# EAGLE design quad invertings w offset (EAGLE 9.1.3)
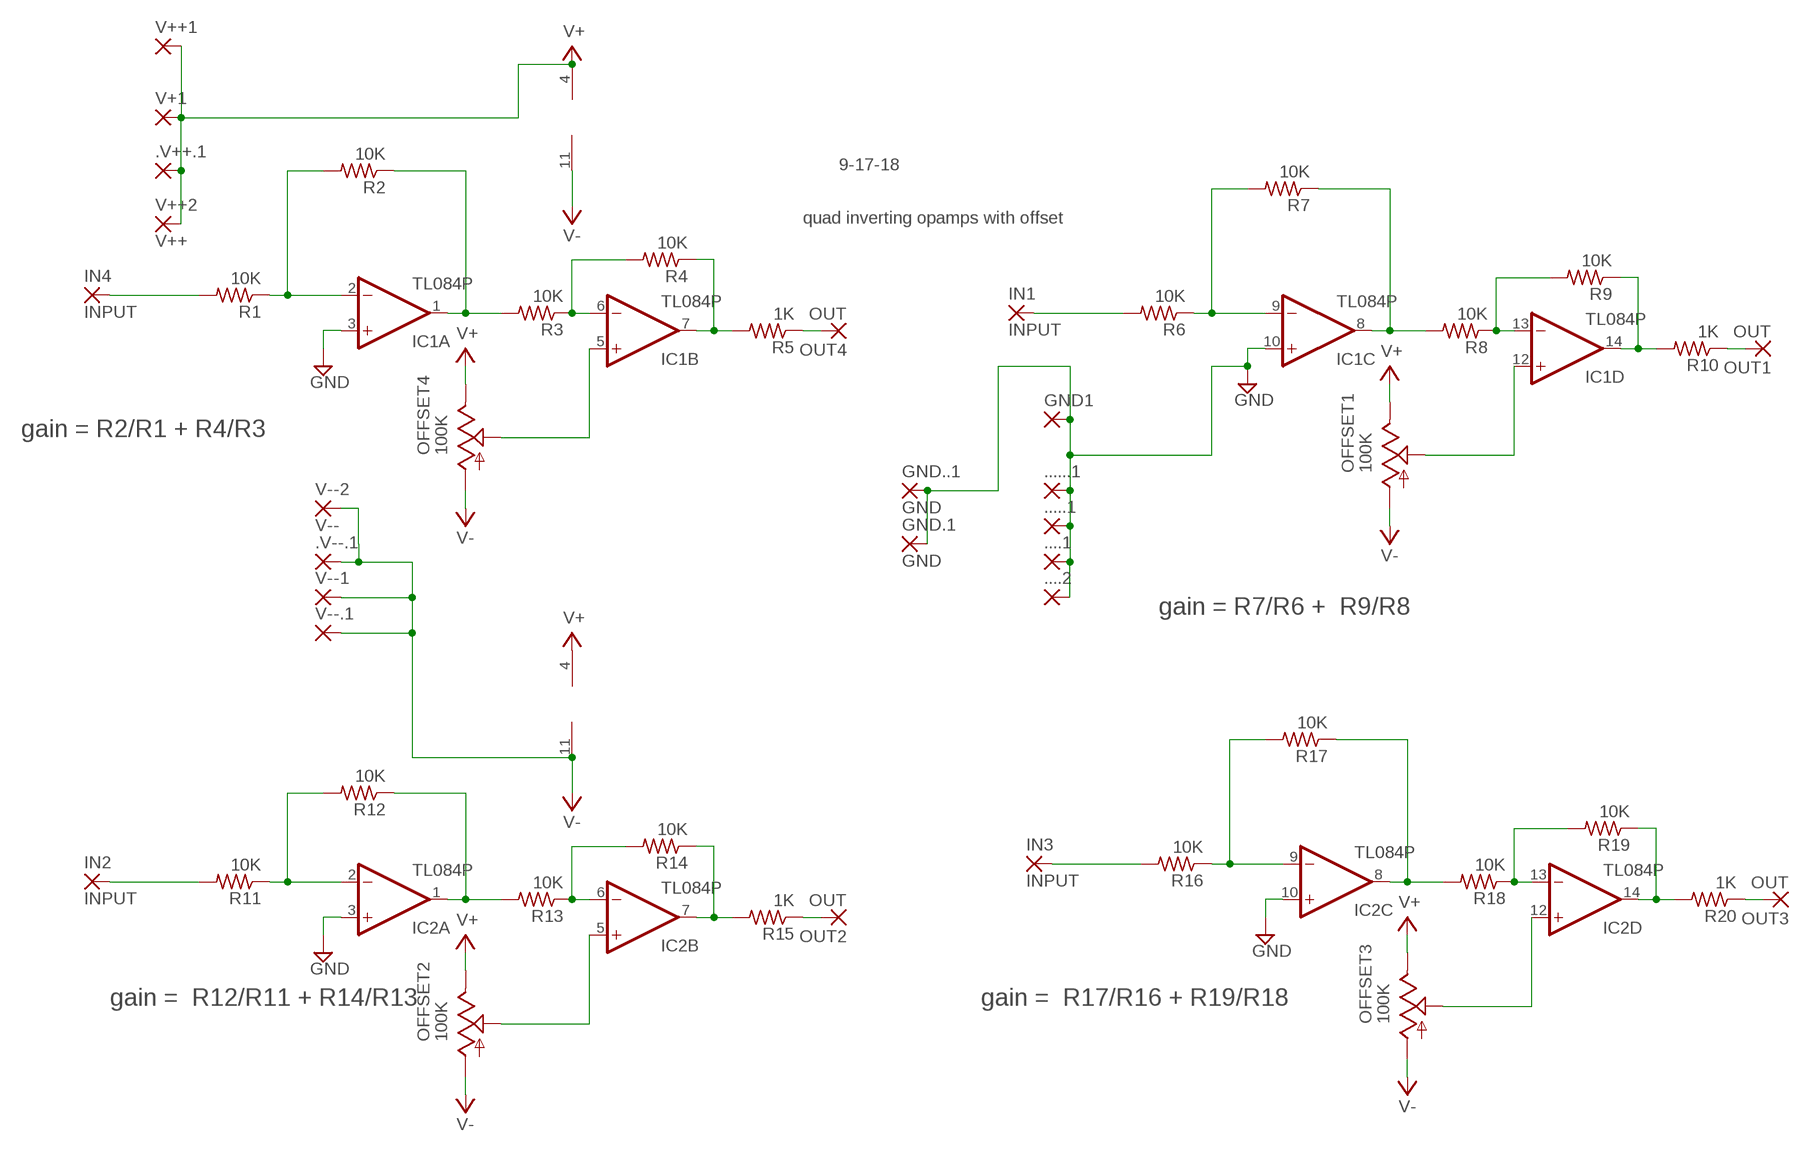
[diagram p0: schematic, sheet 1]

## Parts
....1  3,17/1,3  [3,17/1,3]
....2  3,17/1,3  [3,17/1,3]
.....1  3,17/1,3  [3,17/1,3]
......1  3,17/1,3  [3,17/1,3]
.V++.1  3,17/1,3  [3,17/1,3]
.V--.1  3,17/1,3  [3,17/1,3]
GND1  3,17/1,3  [3,17/1,3]
GND.1  GND  1,6/0,8  [1,6/0,8]
GND..1  GND  1,6/0,8  [1,6/0,8]
IC1  TL084P  [DIL14]
IC2  TL084P  [DIL14]
IN1  INPUT  3,17/1,3  [3,17/1,3]
IN2  INPUT  3,17/1,3  [3,17/1,3]
IN3  INPUT  3,17/1,3  [3,17/1,3]
IN4  INPUT  3,17/1,3  [3,17/1,3]
OFFSET1  100K  TRIM_US-S63X  [S63X]
OFFSET2  100K  TRIM_US-S63X  [S63X]
OFFSET3  100K  TRIM_US-S63X  [S63X]
OFFSET4  100K  TRIM_US-S63X  [S63X]
OUT1  OUT  3,17/1,3  [3,17/1,3]
OUT2  OUT  3,17/1,3  [3,17/1,3]
OUT3  OUT  3,17/1,3  [3,17/1,3]
OUT4  OUT  3,17/1,3  [3,17/1,3]
R1  10K  R-US_0204/7  [0204/7]
R2  10K  R-US_0204/7  [0204/7]
R3  10K  R-US_0204/7  [0204/7]
R4  10K  R-US_0204/7  [0204/7]
R5  1K  R-US_0204/7  [0204/7]
R6  10K  R-US_0204/7  [0204/7]
R7  10K  R-US_0204/7  [0204/7]
R8  10K  R-US_0204/7  [0204/7]
R9  10K  R-US_0204/7  [0204/7]
R10  1K  R-US_0204/7  [0204/7]
R11  10K  R-US_0204/7  [0204/7]
R12  10K  R-US_0204/7  [0204/7]
R13  10K  R-US_0204/7  [0204/7]
R14  10K  R-US_0204/7  [0204/7]
R15  1K  R-US_0204/7  [0204/7]
R16  10K  R-US_0204/7  [0204/7]
R17  10K  R-US_0204/7  [0204/7]
R18  10K  R-US_0204/7  [0204/7]
R19  10K  R-US_0204/7  [0204/7]
R20  1K  R-US_0204/7  [0204/7]
V+1  3,17/1,3  [3,17/1,3]
V++1  3,17/1,3  [3,17/1,3]
V++2  V++  1,6/0,8  [1,6/0,8]
V--1  3,17/1,3  [3,17/1,3]
V--2  V--  1,6/0,8  [1,6/0,8]
V--.1  3,17/1,3  [3,17/1,3]

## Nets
GND: ....1.1(P) ....2.1(P) .....1.1(P) ......1.1(P) GND1.1(P) GND.1.1(P) GND..1.1(P) IC1.3(A:+IN) IC1.10(C:+IN) IC2.3(A:+IN) IC2.10(C:+IN)
N$1: IC1.5(B:+IN) OFFSET4.S
N$2: OUT4.1(P) R5.1
N$3: IN4.1(P) R1.2
N$4: IC1.8(C:OUT) R7.1 R8.2
N$5: IC1.2(A:-IN) R1.1 R2.2
N$6: IC1.6(B:-IN) R3.1 R4.2
N$7: IC1.7(B:OUT) R4.1 R5.2
N$8: IN1.1(P) R6.2
N$9: IC1.9(C:-IN) R6.1 R7.2
N$10: IC1.12(D:+IN) OFFSET1.S
N$11: IC1.13(D:-IN) R8.1 R9.2
N$12: IC1.14(D:OUT) R9.1 R10.2
N$13: OUT1.1(P) R10.1
N$14: IC2.1(A:OUT) R12.1 R13.2
N$15: IN2.1(P) R11.2
N$16: IC2.2(A:-IN) R11.1 R12.2
N$17: IC2.5(B:+IN) OFFSET2.S
N$18: IC1.1(A:OUT) R2.1 R3.2
N$19: IC2.6(B:-IN) R13.1 R14.2
N$20: IC2.7(B:OUT) R14.1 R15.2
N$21: OUT2.1(P) R15.1
N$22: IC2.8(C:OUT) R17.1 R18.2
N$23: IN3.1(P) R16.2
N$24: IC2.9(C:-IN) R16.1 R17.2
N$25: IC2.12(D:+IN) OFFSET3.S
N$26: IC2.13(D:-IN) R18.1 R19.2
N$27: IC2.14(D:OUT) R19.1 R20.2
N$28: OUT3.1(P) R20.1
V+: .V++.1.1(P) IC1.4(P:V+) IC2.4(P:V+) OFFSET1.E OFFSET2.E OFFSET3.E OFFSET4.E V+1.1(P) V++1.1(P) V++2.1(P)
V-: .V--.1.1(P) IC1.11(P:V-) IC2.11(P:V-) OFFSET1.A OFFSET2.A OFFSET3.A OFFSET4.A V--1.1(P) V--2.1(P) V--.1.1(P)

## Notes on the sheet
- 9-17-18
- quad inverting opamps with offset
- gain = R2/R1 + R4/R3
- gain = R7/R6 +  R9/R8
- gain =  R12/R11 + R14/R13 | gain =  R17/R16 + R19/R18

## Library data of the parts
....1 ....2 .....1 ......1 .V++.1 .V--.1 GND1 V+1 V++1 V--1 V--.1 = wirepad-NONAMES:3,17/1,3: THROUGH-HOLE PAD
GND.1 GND..1 V++2 V--2 = wirepad-NONAMES:1,6/0,8: THROUGH-HOLE PAD
IC1 IC2 = linear:TL084: OP AMP
IN1-IN4 OUT1-OUT4 = wirepad:3,17/1,3: THROUGH-HOLE PAD
OFFSET1-OFFSET4 = pot:TRIM_US-: POTENTIOMETER
R1-R20 = rcl:R-US_: RESISTOR, American symbol

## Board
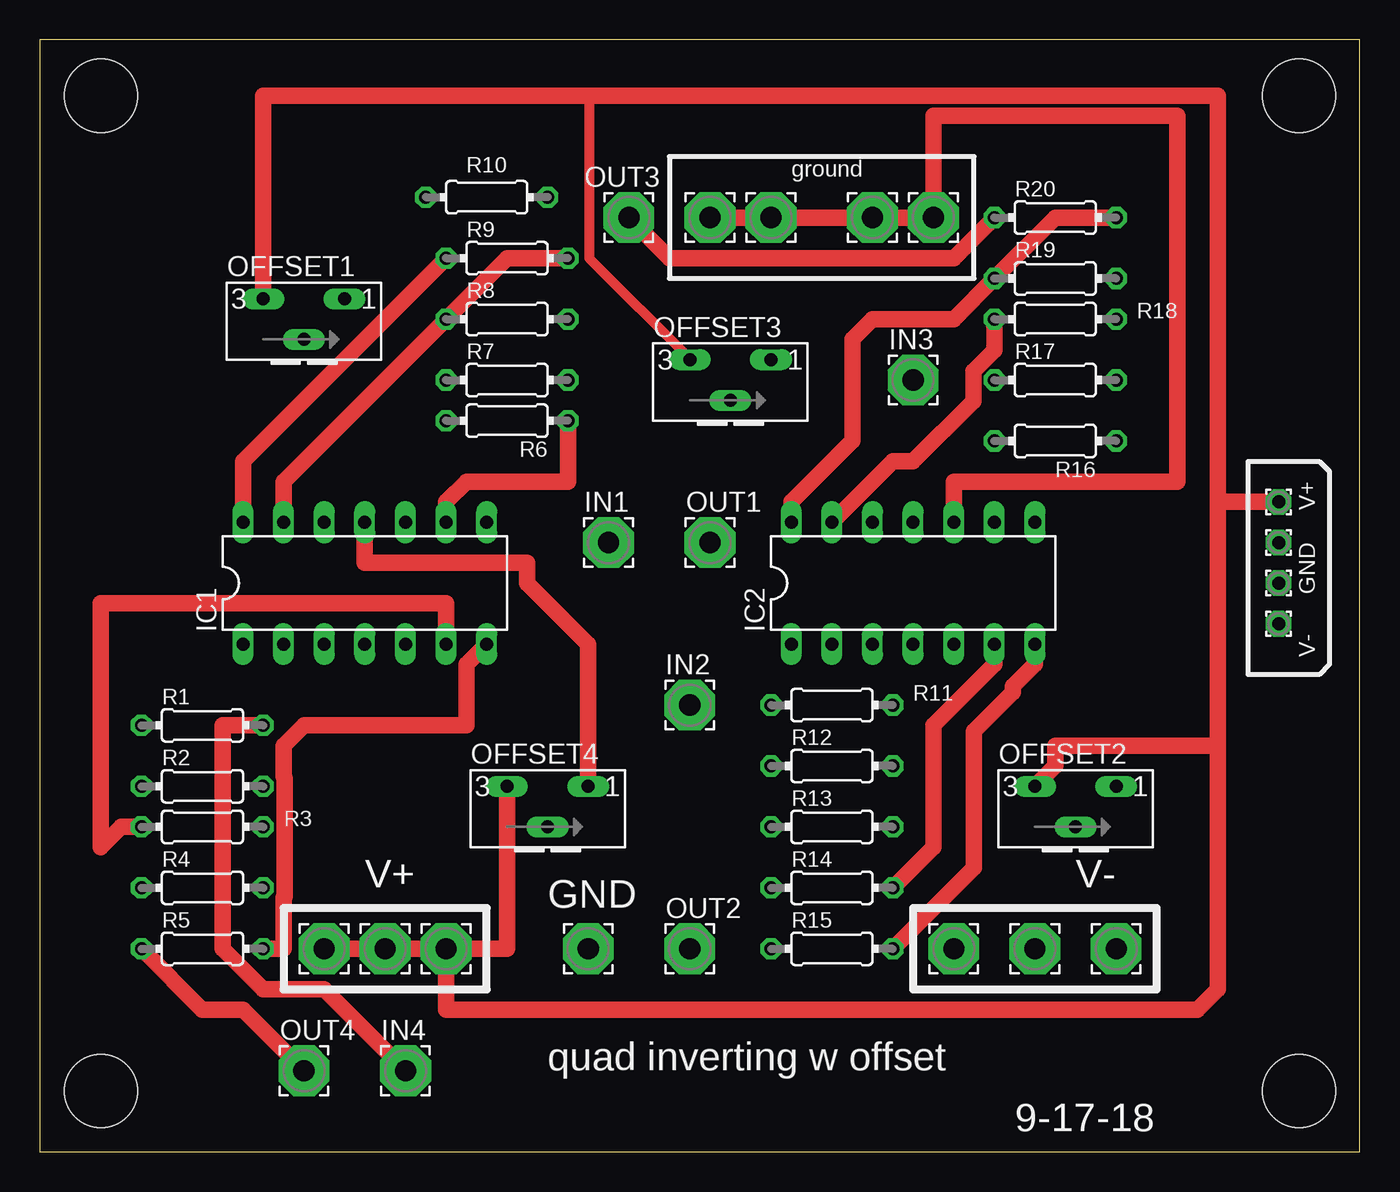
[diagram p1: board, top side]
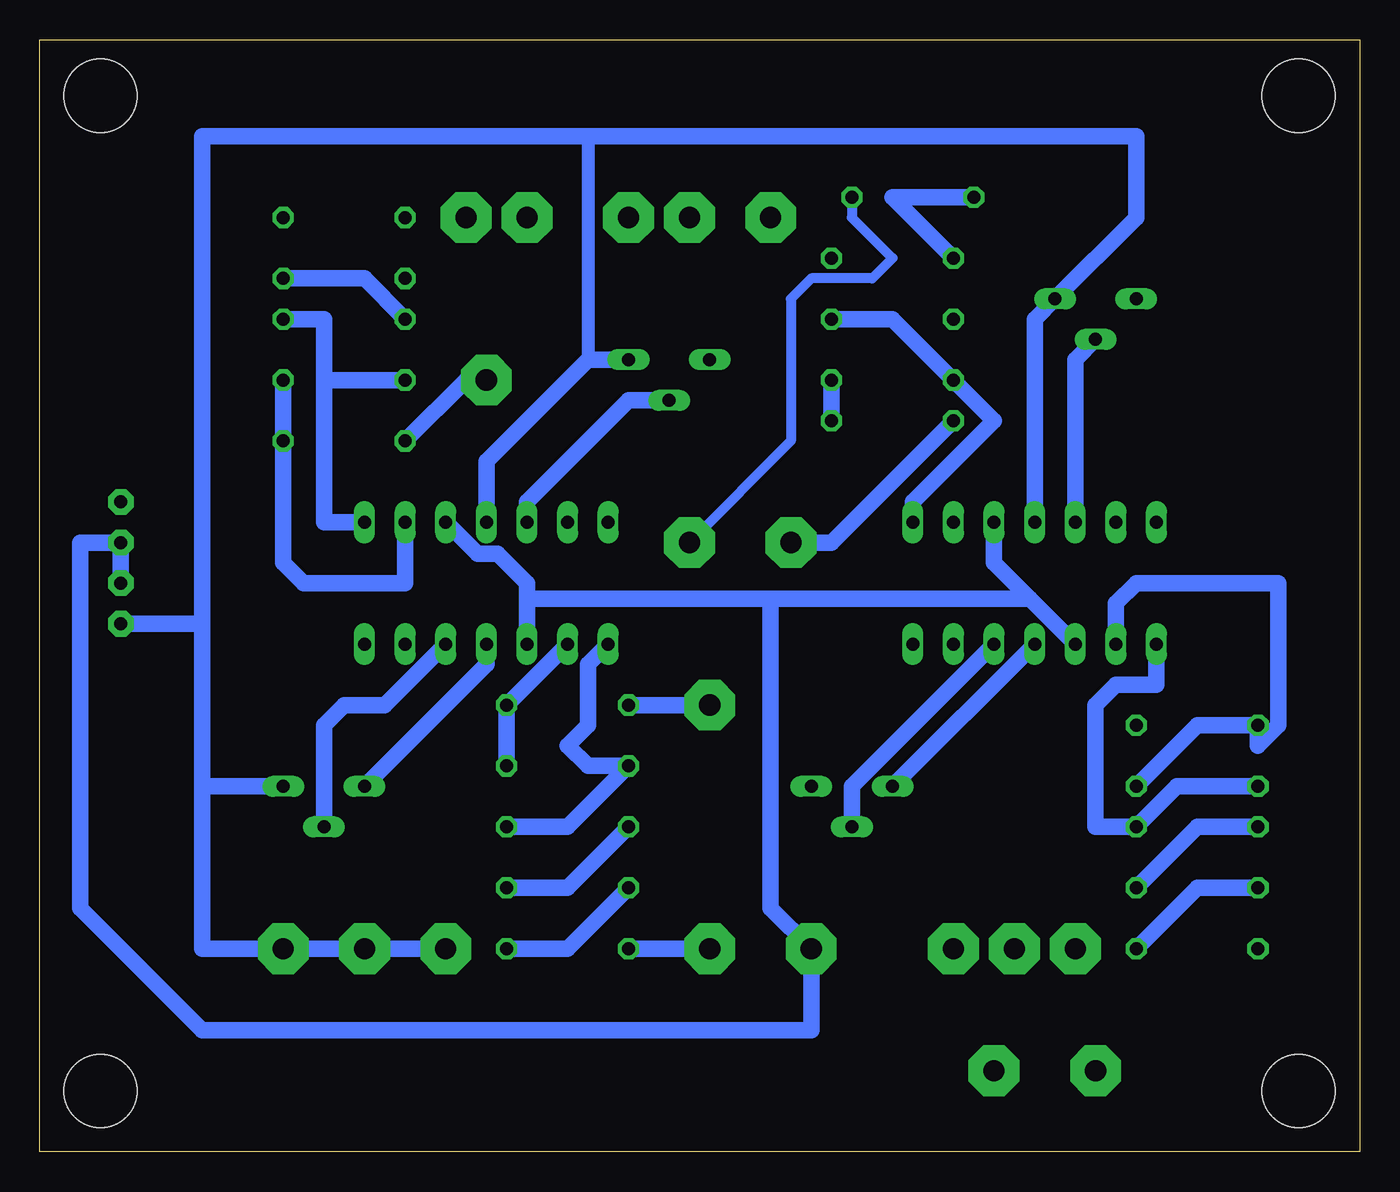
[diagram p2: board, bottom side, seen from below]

Size 82.53 x 69.52 mm. Coordinates in mm from the lower left corner, seen from the top.
Outline: 0,0 82.53,0 82.53,69.52 0,69.52 0,0
Copper layers (1*16): Top 0.035mm / dielectric 1.5mm / Bottom 0.035mm
Design rules "default": minimum track width 6mil, minimum drill 0.35mm, track to track 6mil, track to pad 6mil, pad to pad 6mil, via to via 6mil, smd to smd 6mil, copper to edge 40mil, drill to drill 6mil, minimum pad ring 10mil, minimum via ring 8mil, stop-mask expansion 4mil, vias tented up to drill 0mil, thermal gap 10mil
Holes 4.57 mm at 3.81,66.04 3.81,3.81 78.74,3.81 78.74,66.04

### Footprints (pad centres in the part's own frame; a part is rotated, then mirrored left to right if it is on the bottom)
3,17/1,3 = drill 1.321 pad 3.175 octagon: 1 0,0
1,6/0,8 = drill 0.813 pad 1.6 octagon: 1 0,0
DIL14 = drill 0.813 long: 1 -7.62,-3.81; 2 -5.08,-3.81; 3 -2.54,-3.81; 4 0,-3.81; 5 2.54,-3.81; 6 5.08,-3.81; 7 7.62,-3.81; 8 7.62,3.81; 9 5.08,3.81; 10 2.54,3.81; 11 0,3.81; 12 -2.54,3.81; 13 -5.08,3.81; 14 -7.62,3.81
S63X = drill 0.813 long: A 2.54,0; E -2.54,0; S 0,-2.54
0204/7 = drill 0.813 octagon: 1 -3.81,0; 2 3.81,0

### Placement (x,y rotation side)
....1  45.72,58.42 0 top
....2  34.29,12.7 0 top
.....1  52.07,58.42 0 top
......1  55.88,58.42 0 top
.V++.1  25.4,12.7 0 top
.V--.1  62.23,12.7 0 top
GND1  41.91,58.42 0 top
GND.1  77.47,35.56 0 top
GND..1  77.47,38.1 0 top
IC1  20.32,35.56 0 top
IC2  54.61,35.56 0 top
IN1  35.56,38.1 0 top
IN2  40.64,27.94 0 top
IN3  54.61,48.26 0 top
IN4  22.86,5.08 0 top
OFFSET1  16.51,53.34 0 top
OFFSET2  64.77,22.86 0 top
OFFSET3  43.18,49.53 0 top
OFFSET4  31.75,22.86 0 top
OUT1  41.91,38.1 0 top
OUT2  40.64,12.7 0 top
OUT3  36.83,58.42 0 top
OUT4  16.51,5.08 0 top
R1  10.16,26.67 0 top
R2  10.16,22.86 0 top
R3  10.16,20.32 0 top
R4  10.16,16.51 0 top
R5  10.16,12.7 0 top
R6  29.21,45.72 180 top
R7  29.21,48.26 0 top
R8  29.21,52.07 0 top
R9  29.21,55.88 0 top
R10  27.94,59.69 180 top
R11  49.53,27.94 180 top
R12  49.53,24.13 0 top
R13  49.53,20.32 0 top
R14  49.53,16.51 0 top
R15  49.53,12.7 0 top
R16  63.5,44.45 180 top
R17  63.5,48.26 0 top
R18  63.5,52.07 0 top
R19  63.5,54.61 0 top
R20  63.5,58.42 0 top
V+1  17.78,12.7 0 top
V++1  21.59,12.7 0 top
V++2  77.47,40.64 270 top
V--1  57.15,12.7 0 top
V--2  77.47,33.02 270 top
V--.1  67.31,12.7 0 top

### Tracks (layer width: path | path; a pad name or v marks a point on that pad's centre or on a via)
GND
  Top 1.016: GND1.1 ....1.1 .....1.1 ......1.1 55.88,62.23 55.88,64.77 71.12,64.77 71.12,62.23 71.12,41.91 57.15,41.91 IC2.10
  Bottom 1.016: IC2.3 52.07,34.58 | IC2.10 57.14,39.37 55.16,37.39 53.9,37.39 52.07,35.56 52.07,34.58 | IC1.3 20.61,34.58 | IC1.10 22.86,36.83 20.61,34.58 | 20.61,34.58 36.83,34.58 | 36.83,34.58 52.07,34.58 | 36.83,34.58 36.83,15.24 ....2.1 34.29,7.62 72.39,7.62 80.01,15.24 80.01,38.1 78.56,38.1 GND..1.1 GND.1.1
N$1
  Bottom 1.016: OFFSET4.S 31.75,22.86 IC1.5
N$2
  Top 1.016: R5.1 10.16,8.89 12.7,8.89 OUT4.1
N$3
  Top 1.016: IN4.1 17.78,10.16 13.97,10.16 11.43,12.7 11.43,26.67 R1.2
N$4
  Bottom 1.016: IC1.8 27.94,40.64 22.86,45.72 R7.1 29.21,52.07 R8.2
N$5
  Bottom 1.016: R2.2 10.16,26.67 R1.1 6.35,25.4 5.08,26.67 5.08,35.56 13.97,35.56 15.24,34.29 IC1.2
N$6
  Top 1.016: IC1.6 25.4,34.29 3.81,34.29 3.81,19.05 5.08,20.32 R3.1
  Bottom 1.016: R4.2 10.16,20.32 R3.1
N$7
  Top 1.016: IC1.7 26.67,30.48 26.67,26.67 16.51,26.67 15.24,25.4 15.24,23.46 15.29,23.41 15.29,15.96 15.24,15.91 15.24,12.7 R5.2
  Bottom 1.016: R5.2 10.16,16.51 R4.1
N$8
  Bottom 1.016: R6.2 33.02,38.1 IN1.1
N$9
  Top 1.016: IC1.9 25.4,40.64 26.67,41.91 33.02,41.91 R6.1
  Bottom 1.016: R6.1 R7.2
N$10
  Bottom 1.016: IC1.12 17.78,49.53 OFFSET1.S
N$11
  Top 1.016: R9.2 29.21,55.88 R8.1 15.24,41.91 IC1.13
N$12
  Top 1.016: IC1.14 12.7,43.18 R9.1
  Bottom 1.016: R9.1 29.21,59.69 R10.2
N$13
  Bottom 0.61: R10.1 31.75,58.42 29.21,55.88 30.48,54.61 34.29,54.61 35.56,53.34 35.56,44.45 OUT1.1
N$14
  Bottom 1.016: R13.2 49.53,20.32 R12.1 48.26,24.13 49.53,25.4 48.26,26.67 48.26,30.48 IC2.1
N$15
  Bottom 1.016: R11.2 IN2.1
N$16
  Bottom 1.016: R12.2 R11.1 IC2.2
N$17
  Bottom 1.016: OFFSET2.S 64.77,26.67 63.5,27.94 60.96,27.94 IC2.5
N$18
  Bottom 1.016: R2.1 11.43,22.86 R3.2 16.51,20.32 16.51,27.94 15.24,29.21 12.7,29.21 IC1.1
N$19
  Top 1.016: R14.2 55.88,19.05 55.88,26.67 59.69,30.48 IC2.6
  Bottom 1.016: R14.2 49.53,16.51 R13.1
N$20
  Top 1.016: R15.2 58.42,17.78 58.42,26.29 60.86,28.73 60.86,29.11 62.23,30.48 IC2.7
  Bottom 1.016: R15.2 49.53,12.7 R14.1
N$21
  Bottom 1.016: R15.1 OUT2.1
N$22
  Bottom 1.016: IC2.8 64.77,39.37 64.77,48.26 | 64.77,48.26 R17.1 | 64.77,48.26 64.77,52.07 R18.2
N$23
  Bottom 1.016: R16.2 55.88,48.26 IN3.1
N$24
  Bottom 1.016: IC2.9 59.69,35.56 66.04,35.56 67.31,36.83 R16.1 R17.2
N$25
  Bottom 1.016: IC2.12 52.07,40.64 45.72,46.99 OFFSET3.S
N$26
  Top 1.016: R18.1 59.69,50.13 58.37,48.81 58.37,46.94 54.61,43.18 53.34,43.18 IC2.13
  Bottom 1.016: R19.2 62.23,54.61 R18.1
N$27
  Top 1.016: R20.2 63.5,58.42 R19.1 57.15,52.07 52.07,52.07 50.8,50.8 50.8,44.45 46.99,40.64 IC2.14
N$28
  Top 1.016: OUT3.1 39.37,55.88 57.15,55.88 R20.1
V+
  Top 0.61: 34.29,66.04 34.34,65.99 34.34,55.88 40.64,49.58 OFFSET3.E
  Top 1.016: 73.66,25.4 73.66,10.16 72.39,8.89 25.4,8.89 .V++.1.1 V++1.1 20.32,12.7 | 73.66,25.4 63.5,25.4 63.5,24.13 OFFSET2.E | 73.66,25.4 73.66,26.67 73.66,40.64 | 73.66,40.64 73.66,66.04 36.83,66.04 34.29,66.04 30.48,66.04 13.97,66.04 OFFSET1.E | 20.32,12.7 29.21,12.7 OFFSET4.E | V+1.1 20.32,12.7 | 73.66,40.64 75.15,40.64 V++2.1
  Bottom 1.016: OFFSET4.E IC1.4 | OFFSET2.E 54.61,30.48 IC2.4
V-
  Top 1.016: OFFSET4.A 34.29,31.75 30.48,35.56 30.48,36.83 20.32,36.83 IC1.11
  Bottom 0.813: 48.26,63.5 48.26,49.53
  Bottom 1.016: V--1.1 .V--.1.1 V--.1.1 72.39,12.7 72.39,22.86 | 72.39,22.86 OFFSET2.A | IC1.11 20.32,52.07 OFFSET1.A 13.97,58.42 13.97,63.5 45.72,63.5 48.26,63.5 72.39,63.5 72.39,49.53 72.39,34.29 72.39,33.02 | IC2.11 54.61,43.18 48.26,49.53 OFFSET3.A | 72.39,33.02 V--2.1 | 72.39,22.86 72.39,33.02

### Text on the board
tNames: ground | V+ | GND | V- | V+ | V- | GND | quad inverting w offset | 9-17-18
